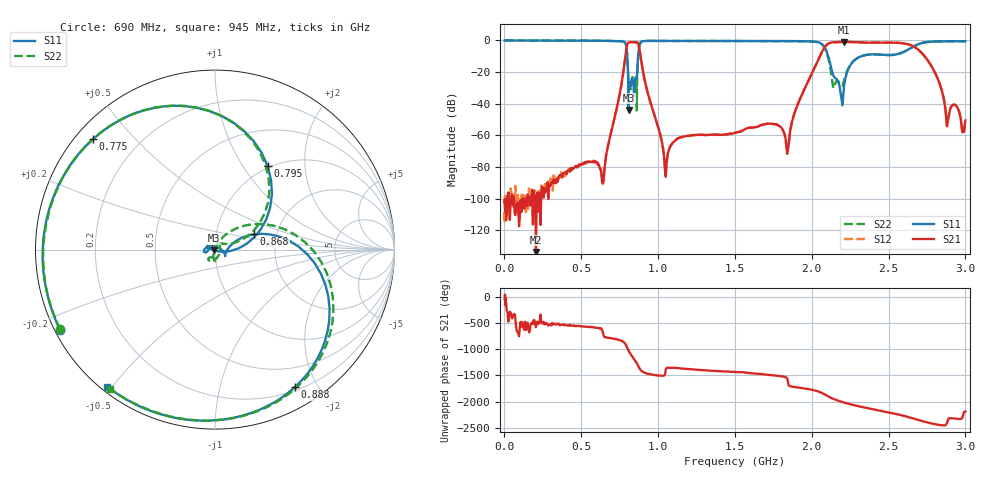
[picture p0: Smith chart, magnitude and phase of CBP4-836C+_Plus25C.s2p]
! Mini-Circuits
! S2P DATA File Format
! Type: BAND PASS FILTER
! Model: CBP4-836C+
! All S Parameters are in dB deg format
! TEST CONDITIONS: INPUT POWER = 0 dBm @ Temperature = +25deg C
! 636 Frequency points
# MHz S DB R 50
!FREQMAG(S11)PHS(S11)MAG(S21)PHS(S21)MAG(S12)PHS(S12)MAG(S22)PHS(S22)
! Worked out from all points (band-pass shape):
!   636 points, 1 MHz to 3 GHz, reference 50 ohm
!   highest |S21| = -0.91 dB at 2.21 GHz (marker M1); lowest = -133.7 dB at 205 MHz (marker M2)
!   |S21| within 3 dB of the highest: 795.5 MHz to 875.4 MHz (79.87 MHz wide, 9.56 % of centre); 2.087 GHz to 2.665 GHz (577.2 MHz wide, 24.3 % of centre)
!   lowest |S11| = -44.0 dB at 808 MHz (marker M3), VSWR 1.01, Z = 49.6 - j0.443 ohm
!   |S11| at or under -10 dB: 799.3 MHz to 869.9 MHz (70.6 MHz wide, 8.46 % of centre); 2.107 GHz to 2.322 GHz (214.8 MHz wide, 9.7 % of centre)
!   |S22| runs from -44.2 to 0.0 dB; largest |S21 - S12| = 0.0087
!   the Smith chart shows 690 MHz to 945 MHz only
!   S11 on the Smith chart (normalised r, x): 690 MHz: 0.01, -0.25; 775 MHz: 0.05, +0.38; 795 MHz: 0.98, +1.30; 868 MHz: 1.53, +0.28; 888 MHz: 0.24, -1.71; 945 MHz: 0.02, -0.49
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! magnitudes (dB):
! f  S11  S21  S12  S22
! 1 MHz  0.0  -101.8  -108.1  0.0
! 205 MHz  0.0  -133.7  -98.0  0.0
! 505 MHz  -0.1  -77.7  -77.9  -0.1
! 640 MHz  -0.2  -90.2  -90.8  -0.2
! 690 MHz  -0.2  -59.7  -59.6  -0.3
! 775 MHz  -0.8  -19.0  -19.0  -0.8
! 795 MHz  -5.2  -4.2  -4.2  -5.1
! 808 MHz  -44.0  -1.3  -1.3  -26.6
! 860 MHz  -24.1  -1.2  -1.2  -33.2
! 868 MHz  -12.6  -1.7  -1.7  -13.5
! 888 MHz  -1.1  -11.5  -11.6  -1.1
! 945 MHz  -0.3  -37.5  -37.5  -0.3
! 1.005 GHz  -0.2  -56.2  -56.2  -0.3
! 1.05 GHz  -0.3  -86.2  -83.5  -0.3
! 1.505 GHz  -0.3  -58.2  -58.3  -0.4
! 1.84 GHz  -0.4  -71.6  -71.6  -0.4
! 2.01 GHz  -0.7  -19.0  -19.0  -0.7
! 2.21 GHz  -28.7  -0.9  -0.9  -25.6
! 2.3 GHz  -11.0  -1.2  -1.2  -11.0
! 2.51 GHz  -9.2  -1.3  -1.3  -9.2
! 2.72 GHz  -1.6  -8.3  -8.3  -1.6
! 3 GHz  -0.5  -50.6  -50.6  -0.6
